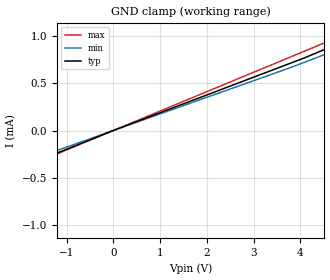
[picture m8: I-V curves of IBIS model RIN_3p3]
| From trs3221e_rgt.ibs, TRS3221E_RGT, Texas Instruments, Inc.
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[Model]   RIN_3p3
Model_type   Input
Vinl = 0.6
Vinh = 2.4
|   typ   min   max
C_comp   1.07pF   0.83pF   1.45pF
[Voltage Range]   3.3   3   3.6
[Temperature Range]   27   110   -40
[Power Clamp Reference]   3.3   3   3.6
[GND Clamp Reference]   0   0   0
[GND Clamp]
|   Voltage   I(typ)   I(min)   I(max)
-25V      -5.173mA   -4.828mA   -5.656mA
-6.641V   -1.353mA   -1.262mA   -1.481mA
-3.868V   -776.6uA   -723.4uA   -850.7uA
-1.186V   -235.8uA   -208.5uA   -243.9uA
-43.29mV  -8.06uA    -7.513uA   -8.819uA
3.622V    682.5uA    637.9uA    745.6uA
5.203V    1.001mA    937uA      1.077mA
5.511V    1.064mA    996.4uA    1.146mA
5.88V     1.14mA     1.067mA    1.23mA
6.108V    1.187mA    1.112mA    1.281mA
25V       5.106mA    4.777mA    5.57mA
